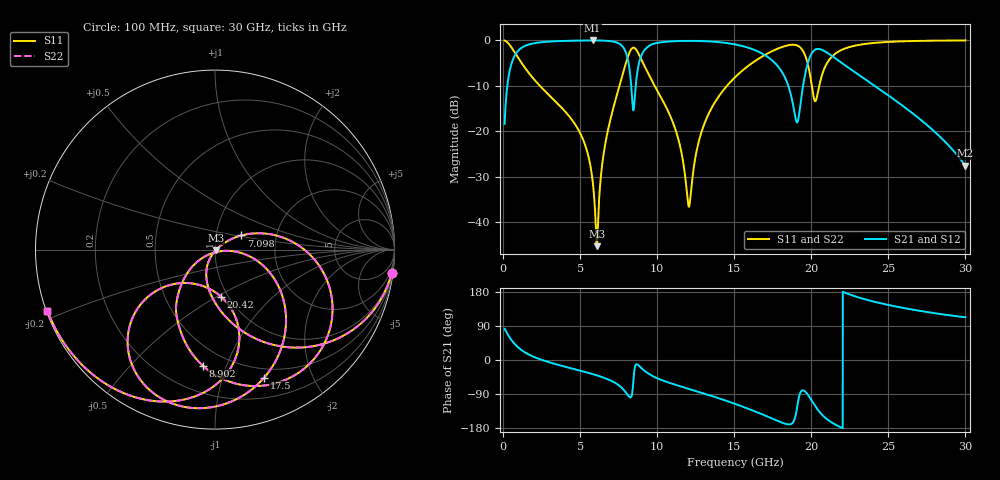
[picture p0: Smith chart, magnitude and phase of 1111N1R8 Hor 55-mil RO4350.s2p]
# GHz S MA R 50
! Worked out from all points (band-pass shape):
!   3201 points, 100 MHz to 30 GHz, reference 50 ohm
!   highest |S21| = -0.05 dB at 5.809 GHz (marker M1); lowest = -27.6 dB at 30 GHz (marker M2)
!   |S21| within 3 dB of the highest: 815.4 MHz to 8.007 GHz (7.191 GHz wide, 163 % of centre); 9.015 GHz to 16.88 GHz (7.864 GHz wide, 60.7 % of centre)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
!   lowest |S11| = -45.2 dB at 6.08 GHz (marker M3), VSWR 1.01, Z = 50.4 - j0.403 ohm
!   |S11| at or under -10 dB: 2.386 GHz to 7.551 GHz (5.165 GHz wide, 104 % of centre); 9.832 GHz to 14.53 GHz (4.7 GHz wide, 38.6 % of centre); 20.03 GHz to 20.52 GHz (483.7 MHz wide, 2.39 % of centre)
!   |S22| runs from -45.2 to -0.1 dB; largest |S21 - S12| = 0
!   S11 on the Smith chart (normalised r, x): 100 MHz: 1, -15; 7.098 GHz: 1.32, +0.21; 8.902 GHz: 0.37, -0.83; 17.5 GHz: 0.40, -1.38; 20.42 GHz: 0.93, -0.52; 30 GHz: 0.00, -0.18
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0.1  0.9927 -7.6  0.1206 82.4  0.1206 82.4  0.9927 -7.6
0.62325  0.7966 -41.4  0.6037 48.5  0.6037 48.5  0.7966 -41.4
1.735156  0.4236 -76.6  0.9043 13.2  0.9043 13.2  0.4236 -76.6
5.089563  0.08901 -117.0  0.9922 -29.1  0.9922 -29.1  0.08901 -117.0
5.809031  0.02879 -118.0  0.9943 -37.2  0.9943 -37.2  0.02879 -118.0
6.08  0.00548 -46.9  0.9939 -40.5  0.9939 -40.5  0.00548 -46.9
7.098469  0.1659 28.3  0.9702 -56.5  0.9702 -56.5  0.1659 28.3
8.210375  0.7372 -27.3  0.4721 -97.9  0.4721 -97.9  0.7372 -27.3
8.481344  0.8287 -58.1  0.1755 -42.7  0.1755 -42.7  0.8287 -58.1
8.901813  0.651 -95.9  0.6298 -18.4  0.6298 -18.4  0.651 -95.9
10.06978  0.267 -134.2  0.9383 -49.4  0.9383 -49.4  0.267 -134.2
11.3125  0.08917 -146.6  0.9788 -67.0  0.9788 -67.0  0.08917 -146.6
12.06  0.01483 -75.0  0.9839 -76.3  0.9839 -76.3  0.01483 -75.0
13.05044  0.1195 -5.7  0.9768 -88.6  0.9768 -88.6  0.1195 -5.7
15.05  0.3919 -28.4  0.8998 -115.7  0.8998 -115.7  0.3919 -28.4
17.49806  0.764 -69.0  0.5927 -155.1  0.5927 -155.1  0.764 -69.0
19.07716  0.8765 -111.4  0.1249 -125.6  0.1249 -125.6  0.8765 -111.4
20.03956  0.3122 -141.3  0.7221 -108.0  0.7221 -108.0  0.3122 -141.3
20.42266  0.2645 -82.6  0.803 -131.2  0.803 -131.2  0.2645 -82.6
22.10453  0.8012 -94.8  0.5438 179.0  0.5438 179.0  0.8012 -94.8
25.01978  0.9588 -126.7  0.2466 145.1  0.2466 145.1  0.9588 -126.7
30  0.9941 -160.0  0.04185 112.8  0.04185 112.8  0.9941 -160.0
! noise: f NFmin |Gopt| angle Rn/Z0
0.1  0.001893  0.9139  2.978  0.004842
3.417  0.01174  0.5485  25.52  0.00443
6.743  0.03427  0.6772  44.31  0.01769
10.06  0.06671  0.7502  65.5  0.03839
13.39  0.05904  0.6543  82.78  0.01893
16.7  0.1081  0.7581  99.27  0.03895
20.03  0.3379  0.8996  117.9  0.1974
23.35  0.1916  0.8164  130.6  0.04002
26.67  0.3171  0.8865  145  0.05676
30  0.9464  0.962  160.9  0.1573
